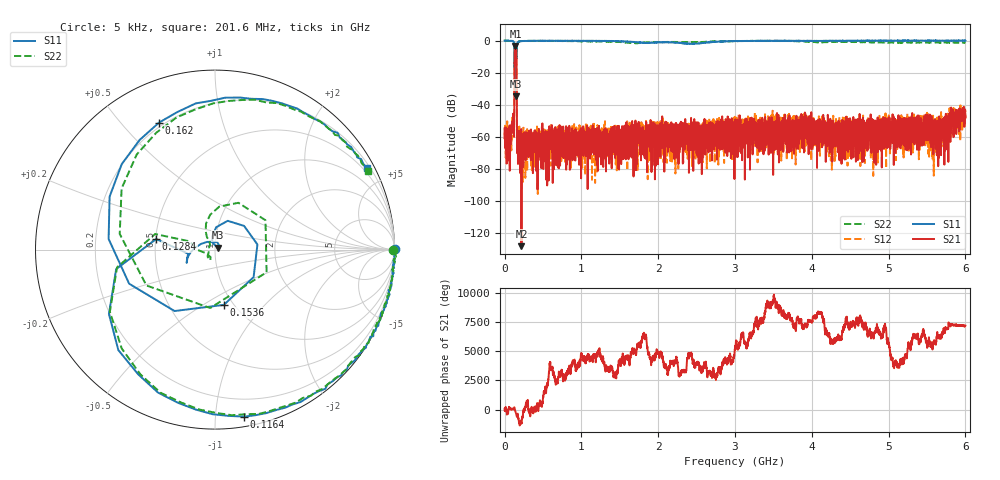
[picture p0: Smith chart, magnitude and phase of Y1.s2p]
#  HZ  S  DB  R  50.00
! Rohde & Schwarz Vector Network Analyzer
! Rohde-Schwarz,ZNL6-2Port,1323001206101378,1.50.1.34-21.10.1.104
! Created: UTC 7/18/2023, 1:59:26 AM
! freq[Hz]  db:S11  ang:S11  db:S21  ang:S21  db:S12  ang:S12  db:S22  ang:S22
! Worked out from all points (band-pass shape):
!   5001 points, 5 kHz to 6 GHz, reference 50 ohm
!   highest |S21| = -3.40 dB at 141.6 MHz (marker M1); lowest = -128.5 dB at 219.6 MHz (marker M2)
!   |S21| within 3 dB of the highest: 131.3 MHz to 152.3 MHz (20.99 MHz wide, 14.8 % of centre)
!   lowest |S11| = -34.7 dB at 142.8 MHz (marker M3), VSWR 1.04, Z = 51.4 + j1.2 ohm
!   |S11| at or under -10 dB: 128.5 MHz to 153.7 MHz (25.18 MHz wide, 17.8 % of centre)
!   |S22| runs from -30.2 to 0.1 dB; largest |S21 - S12| = 0.0089
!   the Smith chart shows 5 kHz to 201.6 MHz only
!   S11 on the Smith chart (normalised r, x): 5 kHz: open; 116.4 MHz: 0.07, -1.19; 128.4 MHz: 0.50, +0.07; 153.6 MHz: 0.90, -0.62; 162 MHz: 0.18, +0.64; 201.6 MHz: 0.34, +3.95
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5000  0.03 0.3  -54.85 64.7  -57.53 -131.8  -0.06 -0.2
4.680496e7  -0.07 -13.2  -54.76 167.5  -66.35 109.8  0.01 -12.9
7.560494e7  -0.02 -25.3  -65.25 62.9  -56.91 84.4  -0.06 -24.1
9.600492e7  -0.14 -41.0  -55.30 64.6  -53.84 58.0  -0.15 -39.9
1.164049e8  -0.50 -80.1  -47.86 9.0  -49.61 13.4  -0.60 -79.2
1.284049e8  -9.55 169.8  -15.55 147.9  -15.62 147.5  -9.26 165.4
1.416049e8  -31.86 29.3  -3.40 170.9  -3.40 170.5  -28.84 156.2
1.428049e8  -34.70 39.3  -3.45 149.2  -3.47 148.8  -28.60 137.7
1.536049e8  -10.12 -81.0  -8.42 -99.1  -8.37 -100.0  -9.75 30.2
1.620049e8  -2.23 113.8  -60.62 85.6  -63.81 122.9  -2.75 116.6
1.872048e8  -0.56 41.0  -61.51 -35.7  -59.29 -63.8  -0.52 39.0
2.016048e8  -0.36 28.2  -56.67 -8.8  -60.79 -28.9  -0.38 27.3
2.196048e8  -0.27 18.8  -128.49 -52.5  -64.66 2.0  -0.28 18.0
4.260046e8  -0.12 -13.6  -63.94 139.4  -60.46 177.1  -0.13 -13.9
1.000804e9  -0.11 -54.5  -58.09 77.1  -54.42 4.0  -0.40 -52.9
2.000403e9  -1.02 -103.6  -60.55 -79.4  -60.54 33.2  -0.95 -95.4
3.000002e9  -0.23 -122.0  -60.17 -121.7  -51.38 -77.8  -0.23 -116.4
4.000802e9  -0.22 -131.6  -59.07 -145.9  -62.14 39.2  -0.78 -126.1
5.000401e9  0.00 -129.4  -55.81 168.8  -55.21 79.2  -1.13 -119.7
5.4372e9  0.04 -126.4  -54.16 84.5  -49.07 -58.6  -1.17 -116.0
5.5932e9  0.01 -126.2  -55.95 129.6  -55.22 108.7  -1.15 -114.9
6e9  -0.02 -122.5  -47.83 -28.4  -43.70 -7.5  -1.31 -111.9
